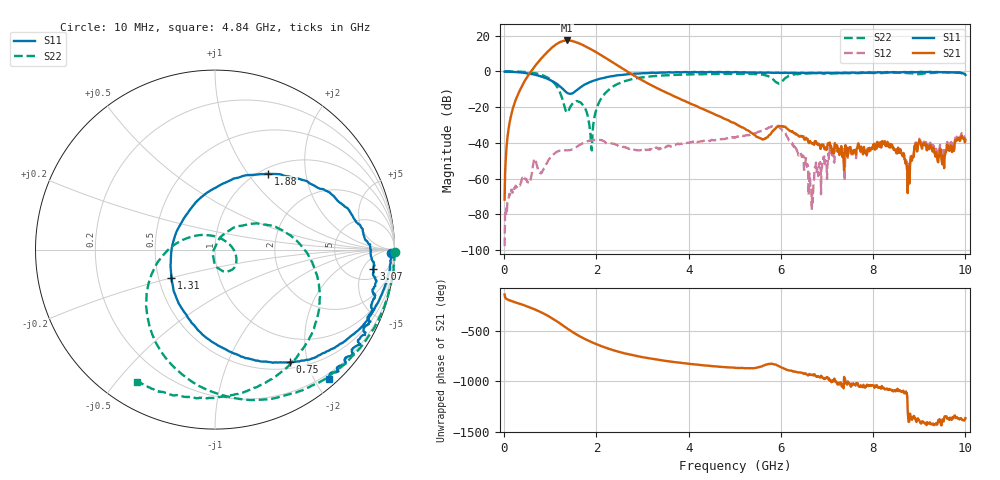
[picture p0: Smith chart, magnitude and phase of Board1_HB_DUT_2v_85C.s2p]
! Created Tue May 27 14:05:12 2025
# hz S ma R 50
! 2 Port Network Data from SP1.SP block
! freq  magS11  angS11  magS21  angS21  magS12  angS12  magS22  angS22
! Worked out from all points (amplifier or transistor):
!   1000 points, 10 MHz to 10 GHz, reference 50 ohm
!   highest |S21| = 17.3 dB at 1.36 GHz (marker M1)
!   |S21| within 3 dB of that: 1.084 GHz to 1.74 GHz (656.7 MHz wide, 46.5 % of centre)
!   unconditionally stable (mu >= 1): 58.14 MHz to 62.67 MHz; 89.37 MHz to 102.8 MHz; 116.7 MHz to end of sweep
!   at 1.67 GHz: K = 8.11, MAG = 15.9 dB, |S12| = -40.7 dB
!   at 5.01 GHz: K = 21.05, MAG = -12.4 dB, |S12| = -36.9 dB
!   at 10 GHz: K = 327.04, MAG = -28.9 dB, |S12| = -36.9 dB
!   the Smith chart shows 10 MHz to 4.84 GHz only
!   S11 on the Smith chart (normalised r, x): 10 MHz: 53, -46; 750 MHz: 0.59, -1.71; 1.31 GHz: 0.58, -0.20; 1.88 GHz: 1.09, +1.25; 3.07 GHz: 8, -8; 4.84 GHz: 0.12, -2.21
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1e7  0.9787 -1.1  0.0002567 -144.8  1.275e-05 -39.1  1.006 -0.8
2e8  0.9635 -13.9  0.102 145.5  0.0005332 77.6  0.9956 -18.4
7.5e8  0.7539 -56.4  1.889 50.7  0.001641 70.3  0.8425 -80.8
9.3e8  0.6287 -74.2  3.434 10.3  0.002757 116.4  0.6851 -110.7
1.09e9  0.495 -95.3  5.266 -32.8  0.005001 101.6  0.4644 -145.3
1.19e9  0.3972 -113.6  6.402 -63.1  0.00591 88.2  0.2911 -173.7
1.31e9  0.2883 -147.3  7.245 -101.6  0.00615 76.1  0.1032 127.5
1.36e9  0.2524 -167.4  7.344 -117.5  0.006123 74.5  0.06995 70.8
1.51e9  0.2541 126.8  6.89 -162.5  0.006964 74.7  0.1357 -29.2
1.68e9  0.375 81.8  5.665 153.1  0.009332 66.9  0.1264 -70.4
1.88e9  0.5154 55.0  4.183 108.6  0.01163 46.6  0.01168 -139.7
2.24e9  0.6949 28.5  2.211 44.5  0.009751 11.8  0.2819 31.0
2.58e9  0.8068 10.7  1.166 -1.7  0.007663 1.4  0.5164 -2.5
3.07e9  0.8889 -7.0  0.4971 -48.8  0.006312 11.0  0.6999 -37.5
3.34e9  0.9168 -15.6  0.3266 -68.8  0.006747 10.3  0.7538 -52.9
4.84e9  0.9615 -48.6  0.04376 -142.6  0.0135 -9.8  0.8541 -120.5
5.01e9  0.9592 -52.1  0.03454 -147.9  0.01425 -12.6  0.8553 -126.9
5.95e9  0.9107 -72.1  0.02979 -129.5  0.02927 -100.6  0.455 -150.3
6.67e9  0.8975 -92.6  0.009555 142.2  0.0001324 1.5  0.8976 -157.7
8.34e9  0.9319 -135.1  0.007543 -7.2  0.007849 -11.8  0.9142 166.9
8.75e9  0.9477 -142.4  0.0003903 148.1  0.0004615 134.5  0.9005 158.6
1e10  0.7999 -161.6  0.012 75.9  0.01425 71.3  0.8308 145.2
